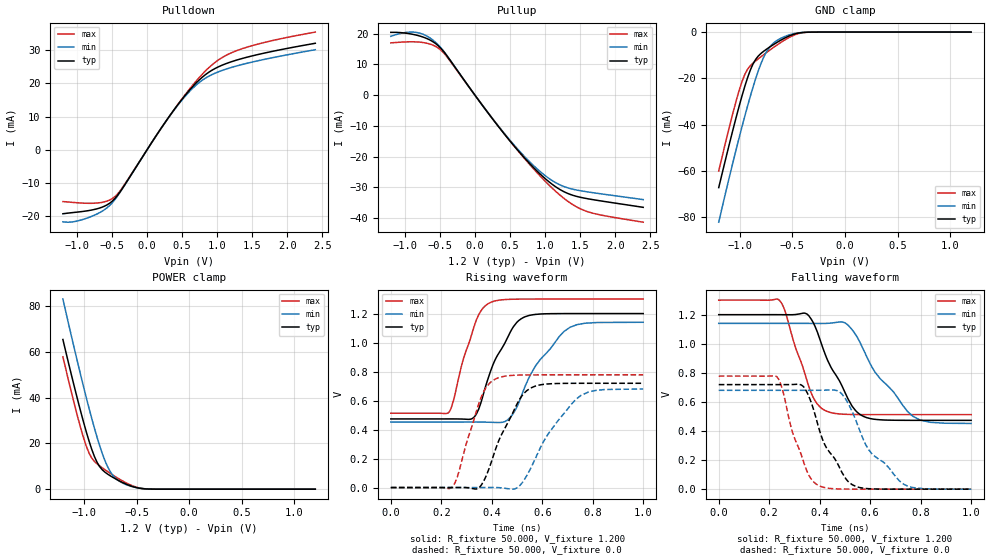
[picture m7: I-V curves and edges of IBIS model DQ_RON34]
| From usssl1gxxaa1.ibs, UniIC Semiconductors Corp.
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|   Model DQ_RON34
[Model] DQ_RON34
Model_type I/O
Vinl =  0.500V
Vinh =  0.700V
Vmeas =  0.600V
Rref =  50.000
Vref =  0.600V
C_comp   1.373pF   1.353pF   1.403pF
[Model Spec]
Vinh   0.700V   0.670V   0.750V
Vinl   0.500V   0.470V   0.550V
Vmeas   0.600V   0.570V   0.650V
Vref   0.600V   0.570V   0.650V
Rref   50.000   NA   NA
[Temperature Range]   25.000   0.125k   -40.000
[Voltage Range]   1.200V   1.140V   1.300V
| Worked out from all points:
|   slope of the pulldown table from 0 to 0.18 V, typ, clamps not added: 30.8 ohm
|   slope of the pullup table from 0 to 0.18 V, typ, clamps not added: 32.3 ohm
|   GND clamp passes 1 mA (typ) near -0.49 V on its own axis
|   POWER clamp passes 1 mA (typ) near -0.53 V on its own axis
|   rising waveform, R_fixture 50.000, V_fixture 1.200: 20-80 % time 106ps typ, 143ps min, 78.3ps max; typ from 0.473 V to 1.2 V
|   rising waveform, R_fixture 50.000, V_fixture 0.0: 20-80 % time 108ps typ, 146ps min, 80.7ps max; typ from 0 V to 0.719 V
|   falling waveform, R_fixture 50.000, V_fixture 1.200: 20-80 % time 117ps typ, 163ps min, 88.1ps max; typ from 1.2 V to 0.473 V
|   falling waveform, R_fixture 50.000, V_fixture 0.0: 20-80 % time 109ps typ, 153ps min, 81ps max; typ from 0.719 V to 0 V
[Pulldown]
|Voltage   I(typ)   I(min)   I(max)
-1.2V     -19.25mA   -21.68mA   -15.59mA
-1.015V   -18.8mA    -21.53mA   -15.91mA
-756mV    -17.99mA   -19.74mA   -16.08mA
-571mV    -16.59mA   -17.46mA   -15.44mA
-460mV    -14.71mA   -15.03mA   -14.13mA
-349mV    -11.55mA   -11.65mA   -11.33mA
354mV     11.15mA    11.06mA    11.15mA
613mV     18.14mA    17.72mA    18.48mA
798mV     22.05mA    21.11mA    22.99mA
1.02V     25.02mA    23.51mA    27.1mA
1.279V    27.04mA    25.27mA    29.87mA
2.4V      32.1mA     30.16mA    35.47mA
[Pullup]
|Voltage   I(typ)   I(min)   I(max)
-1.2V     20.45mA    19.16mA    17.03mA
-1.004V   20.23mA    20.35mA    17.32mA
-819mV    19.45mA    20.35mA    17.32mA
-634mV    17.86mA    18.51mA    16.59mA
-486mV    15.25mA    15.42mA    14.68mA
106mV     -3.309mA   -3.285mA   -3.265mA
513mV     -15.28mA   -15.03mA   -15.28mA
846mV     -23.8mA    -23.14mA   -24.23mA
1.142V    -29.68mA   -28.36mA   -31.12mA
1.364V    -32.35mA   -30.43mA   -35.17mA
1.586V    -33.63mA   -31.41mA   -37.76mA
2.4V      -36.51mA   -34mA      -41.35mA
[GND_clamp]
|Voltage   I(typ)   I(min)   I(max)
-1.2V     -67.26mA   -82.22mA   -60.1mA
-1.05V    -39.62mA   -53.62mA   -32.4mA
-1V       -31.05mA   -44.64mA   -24.37mA
-950mV    -23.16mA   -36.01mA   -18.1mA
-925mV    -19.62mA   -31.85mA   -16.02mA
-875mV    -13.89mA   -23.97mA   -13.48mA
-800mV    -9.288mA   -13.81mA   -10.72mA
-750mV    -7.535mA   -8.829mA   -8.993mA
-675mV    -5.274mA   -4.578mA   -6.506mA
-525mV    -1.587mA   -1.138mA   -2.208mA
-375mV    -90.13uA   -87.27uA   -132.9uA
1.2V      0A         0A         0A
[POWER_clamp]
|Voltage   I(typ)   I(min)   I(max)
-1.2V     65.51mA    83.21mA    57.91mA
-1.05V    37.38mA    53.57mA    29.99mA
-1V       28.74mA    44.18mA    21.95mA
-950mV    20.85mA    35.16mA    15.65mA
-925mV    17.34mA    30.84mA    13.56mA
-875mV    11.74mA    22.7mA     11.06mA
-800mV    7.436mA    12.47mA    8.502mA
-750mV    5.864mA    7.69mA     6.933mA
-675mV    3.901mA    3.837mA    4.735mA
-525mV    971.5uA    903.1uA    1.25mA
-400mV    85.95uA    125.9uA    91.19uA
1.2V      0A         0A         0A
[Ramp]
| variable   typ   min   max
dV/dt_r   0.431/0.108n   0.408/0.146n   0.466/80.781p
dV/dt_f   0.436/0.117n   0.413/0.162n   0.472/87.928p
R_load = 50.000
[Rising Waveform]
R_fixture= 50.000
V_fixture= 1.200
V_fixture_min= 1.140
V_fixture_max= 1.300
|time   V(typ)   V(min)   V(max)
0s        473.3mV    451.6mV    512.6mV
232ps     473.4mV    451.6mV    523.2mV
331ps     487.7mV    451.8mV    1.117V
356ps     579.4mV    451.6mV    1.216V
393ps     791.3mV    450.3mV    1.275V
462ps     1.032V     465.3mV    1.298V
506ps     1.151V     580.6mV    1.299V
574ps     1.194V     840.4mV    1.3V
710ps     1.2V       1.105V     1.3V
1ns       1.2V       1.14V      1.3V
[Rising Waveform]
R_fixture= 50.000
V_fixture= 0.0
V_fixture_min= 0.0
V_fixture_max= 0.0
|time   V(typ)   V(min)   V(max)
0s        35.08nV    603.6nV    20.74nV
244ps     132.3uV    -8.965uV   5.093mV
265ps     422.7uV    -23.33uV   81.16mV
353ps     4.683mV    229.8uV    600.6mV
417ps     274.1mV    296.5uV    750.9mV
500ps     575.8mV    -2.279mV   775.3mV
554ps     686.2mV    131.8mV    777mV
619ps     714.2mV    358mV      777.3mV
754ps     719.1mV    636.3mV    777.4mV
1ns       719.2mV    679.8mV    777.4mV
[Falling Waveform]
R_fixture= 50.000
V_fixture= 1.200
V_fixture_min= 1.140
V_fixture_max= 1.300
|time   V(typ)   V(min)   V(max)
0s        1.2V       1.14V      1.3V
240ps     1.2V       1.14V      1.3V
350ps     1.204V     1.14V      744mV
382ps     1.118V     1.14V      606.9mV
422ps     926.2mV    1.14V      540.4mV
500ps     666mV      1.144V     515mV
575ps     499.1mV    953.5mV    512.8mV
620ps     480.1mV    803.1mV    512.7mV
769ps     473.4mV    501.4mV    512.6mV
1ns       473.3mV    451.8mV    512.6mV
[Falling Waveform]
R_fixture= 50.000
V_fixture= 0.0
V_fixture_min= 0.0
V_fixture_max= 0.0
|time   V(typ)   V(min)   V(max)
0s        719.2mV    679.9mV    777.4mV
230ps     719.1mV    679.9mV    773.5mV
293ps     719.7mV    679.8mV    387.4mV
337ps     702.3mV    679.7mV    182.8mV
401ps     393.9mV    680.1mV    20.77mV
483ps     132.9mV    662.8mV    1.112mV
544ps     18.22mV    470.6mV    122.9uV
593ps     3.311mV    273.9mV    21.1uV
733ps     25.1uV     33.75mV    149.1nV
1ns       33.66nV    9.973uV    17.71nV
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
